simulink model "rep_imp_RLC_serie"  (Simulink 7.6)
settings: Solver=ode23t  StartTime=0.0  StopTime=0.04  RelTol=1e-3
InitFcn:
  | R=4;
  | C=0.001;
  | L=10e-3;
StopFcn:
  | load UI_RLC_espace_etat.mat
  | subplot 211
  | plot(x(1,:),x(2,:),x(1,:),x(3,:))
  | grid
  | %axis([0 0.04 -0.2 1.2])
  | title('U-I Circuit RLC')
  | xlabel('temps')
  | 
  | subplot 212
  | plot(x(1,:),x(4,:),x(1,:),x(5,:))
  | title('U-I Espace d''état')
  | grid
  | xlabel('temps')
libraries: powerlib x9, powerlib_extras x1

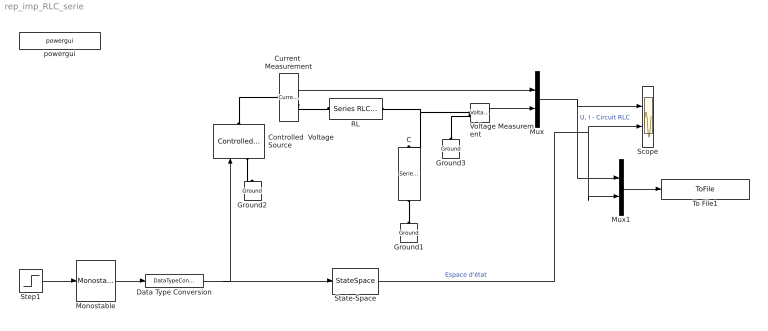
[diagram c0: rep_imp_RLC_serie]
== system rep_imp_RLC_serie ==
  C : powerlib/Elements/Series RLC Branch  DialogController=POWERSYS.PowerSysDialog  PhysicalDomain=powersysdomain  SubClassName=unknown  LeftPortType=p1  RightPortType=p1  LConnTagsString=__new0  RConnTagsString=__new0  BranchType=C  Resistance=1  Inductance=1e-3  SetiL0=off  InitialCurrent=0  Capacitance=0.001  Setx0=off  InitialVoltage=0  Measurements=None
  Controlled  Voltage Source : powerlib/Electrical Sources/Controlled Voltage Source  DialogController=POWERSYS.PowerSysDialog  SystemSampleTime=-1  Initialize=on  Source_Type=AC  Amplitude=0  Phase=0  Frequency=0  Measurements=None
  Current  Measurement : powerlib/Measurements/Current Measurement  DialogController=POWERSYS.PowerSysDialog  SystemSampleTime=-1  PhasorSimulation=off  OutputType=Complex  PSBequivalent=0
  Data Type Conversion : DataTypeConversion  OutDataTypeStr=double
  Ground1 : powerlib/Elements/Ground  DialogController=POWERSYS.PowerSysDialog  PhysicalDomain=powersysdomain  SubClassName=unknown  LeftPortType=p1  RightPortType=p1  LConnTagsString=a
  Ground2 : powerlib/Elements/Ground  DialogController=POWERSYS.PowerSysDialog  PhysicalDomain=powersysdomain  SubClassName=unknown  LeftPortType=p1  RightPortType=p1  LConnTagsString=a
  Ground3 : powerlib/Elements/Ground  DialogController=POWERSYS.PowerSysDialog  PhysicalDomain=powersysdomain  SubClassName=unknown  LeftPortType=p1  RightPortType=p1  LConnTagsString=a
  Monostable : powerlib_extras/Control  Blocks/Monostable  DialogController=POWERSYS.PowerSysDialog  SystemSampleTime=-1  EdgeDetect=Either  t_mono=0.01  ic=0
  Mux : Mux  Inputs=2
  Mux1 : Mux  Inputs=2
  RL : powerlib/Elements/Series RLC Branch  DialogController=POWERSYS.PowerSysDialog  PhysicalDomain=powersysdomain  SubClassName=unknown  LeftPortType=p1  RightPortType=p1  LConnTagsString=__new0  RConnTagsString=__new0  BranchType=RL  Resistance=4  Inductance=10e-3  SetiL0=off  InitialCurrent=0  Capacitance=0  Setx0=off  InitialVoltage=0  Measurements=None
  Scope : Scope  NumInputPorts=2
  State-Space : StateSpace  A=[0 1/C;-1/L -R/L]  B=[0 1/L]'  C=eye(2)  D=[0 0]'
  Step1 : Step  Time=0.01  SampleTime=0
  To File1 : ToFile  Filename=UI_RLC_espace_etat  MatrixName=x
  Voltage Measurement : powerlib/Measurements/Voltage Measurement  DialogController=POWERSYS.PowerSysDialog  SystemSampleTime=-1  PhasorSimulation=off  OutputType=Complex  PSBequivalent=0
  powergui : powerlib/powergui  Priority=1  SystemSampleTime=-1  SimulationMode=Continuous  SampleTime=50e-6  frequency=60  SPID=off  DisableSnubberDevices=off  DisableRonSwitches=off  DisableVfSwitches=off  SwTol=0  Interpol=off  frequencyindice=0  echomessages=off  HookPort=off  DisplayEquations=off  FunctionMessages=off  EnableUseOfTLC=off  x0status=blocks  RestoreLinks=warning  ResistiveCurrentMeasurement=off  Ylog=off  Xlog=on  ShowGrid=off  save=off  variable=ZData  ZoomFFT=off  StartTime=0.0  cycles=1  DisplayStyle=1  fundamental=60  FreqAxis=off  MaxFrequency=1000  frequencyindicesteady=1  display=off  methode=off
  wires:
  Voltage Measurement/1 -> Mux/2
  Current  Measurement/1 -> Mux/1
  Mux/1 -> Scope/1, Mux1/1  "U, I - Circuit RLC"
  Step1/1 -> Monostable/1
  Monostable/1 -> Data Type Conversion/1
  State-Space/1 -> Scope/2, Mux1/2  "Espace d'état"
  Data Type Conversion/1 -> State-Space/1, Controlled  Voltage Source/1
  Mux1/1 -> To File1/1
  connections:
  Current  Measurement/RConn1 -- RL/LConn1
  Voltage Measurement/LConn1 -- RL/RConn1 -- C/LConn1
  C/RConn1 -- Ground1/LConn1
  Controlled  Voltage Source/RConn1 -- Current  Measurement/LConn1
  Controlled  Voltage Source/LConn1 -- Ground2/LConn1
  Ground3/LConn1 -- Voltage Measurement/LConn2
